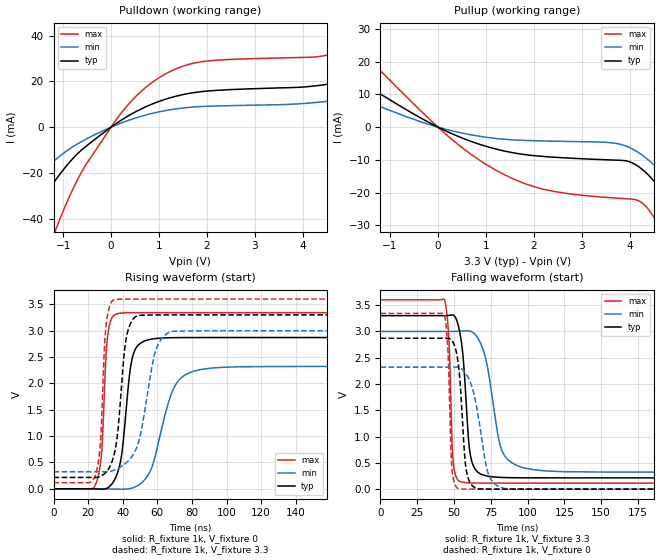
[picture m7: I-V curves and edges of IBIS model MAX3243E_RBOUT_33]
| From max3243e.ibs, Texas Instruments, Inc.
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[Model]   MAX3243E_RBOUT_33
Model_type  Output
Vref =   0
Rref =   3000
Cref =   150p
Vmeas =   1.5
| variable   typ   min   max
C_comp   4.21pF   3.18pF   6.18pF
| C_pullup   3.97pF   3.18pF   5.18pF
| C_pulldown   4.44pF   3.29pF   6.18pF
[Temperature Range]   40   100   -40
| Ambient temperature   25   85   -40
[Voltage range]   3.3   3   3.6
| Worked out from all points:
|   slope of the pulldown table from 0 to 0.495 V, typ, clamps not added: 75.9 ohm
|   slope of the pullup table from 0 to 0.495 V, typ, clamps not added: 152 ohm
|   rising waveform, R_fixture 1k, V_fixture 0: 20-80 % time 5.45ns typ, 11.3ns min, 2.9ns max; typ from 0 V to 2.87 V
|   falling waveform, R_fixture 1k, V_fixture 3.3: 20-80 % time 4.69ns typ, 9.47ns min, 2.43ns max; typ from 3.3 V to 0.215 V
|   rising waveform, R_fixture 1k, V_fixture 3.3: 20-80 % time 5.08ns typ, 8.91ns min, 2.91ns max; typ from 0.215 V to 3.3 V
|   falling waveform, R_fixture 1k, V_fixture 0: 20-80 % time 4.16ns typ, 8.6ns min, 2.22ns max; typ from 2.87 V to 0 V
[Pulldown]
| MAX3243E_RBOUT_33
|   Voltage   I(typ)   I(min)   I(max)
-3.3V     -113.4mA   -74.18mA   -190mA
-2.415V   -70.58mA   -44.83mA   -126.3mA
-1.81V    -45.3mA    -28.2mA    -84.59mA
-1.175V   -23.63mA   -14.52mA   -45.99mA
-595mV    -9.62mA    -6.087mA   -18.88mA
200mV     2.877mA    1.713mA    5.857mA
705mV     8.707mA    5.186mA    17.04mA
1.335V    13.41mA    7.923mA    25.3mA
2.01V     15.77mA    9.121mA    28.89mA
4.405V    18.41mA    11.05mA    31.05mA
6.135V    26.75mA    17.02mA    43.3mA
6.6V      29.92mA    19.27mA    48.02mA
[Pullup]
| MAX3243E_RBOUT_33
|   Voltage   I(typ)   I(min)   I(max)
-3.3V     30.08mA    19.81mA    47.96mA
-2.18V    19.23mA    12.28mA    31.63mA
335mV     -2.284mA   -1.265mA   -4.285mA
1.66V     -8.06mA    -3.97mA    -16.36mA
2.54V     -9.29mA    -4.322mA   -19.92mA
3.89V     -10.22mA   -5.614mA   -21.83mA
4.205V    -12.28mA   -7.993mA   -22.63mA
4.46V     -15.74mA   -10.94mA   -26.56mA
4.625V    -18.71mA   -13.31mA   -30.76mA
5.14V     -31.25mA   -22.85mA   -49.93mA
5.47V     -41.58mA   -30.54mA   -65.91mA
6.6V      -87.28mA   -64.61mA   -134mA
[Ramp]
| MAX3243E_RBOUT_33
| variable   typ   min   max
dV/dt_r   1.73/5.46E-09   1.40/1.14E-08   2.01/2.91E-09
dV/dt_f   1.86/4.72E-09   1.61/9.50E-09   2.10/2.45E-09
R_load = 1k
[Rising Waveform]
| MAX3243E_RBOUT_33
R_fixture =   1k
C_fixture =   0
L_fixture =   0
V_fixture =   0
V_fixture_min = 0
V_fixture_max = 0
|   Time   V(typ)   V(min)   V(max)
0s        331.6pV    2.084nV    131.1pV
24.9ns    -3.34mV    12.77uV    132.3mV
27.9ns    -6.992mV   80.13uV    738.9mV
31.2ns    16.85mV    -1.213mV   2.874V
36.2ns    234.8mV    -5.782mV   3.314V
45.3ns    2.449V     12.87mV    3.341V
53.4ns    2.814V     200.5mV    3.342V
69.2ns    2.867V     1.889V     3.342V
81.2ns    2.87V      2.233V     3.342V
269.9ns   2.87V      2.321V     3.342V
[Falling Waveform]
| MAX3243E_RBOUT_33
R_fixture =   1k
C_fixture =   0
L_fixture =   0
V_fixture =   3.3
V_fixture_min = 3
V_fixture_max = 3.6
|   Time   V(typ)   V(min)   V(max)
0s        3.3V       3V         3.6V
43.6ns    3.3V       3V         3.597V
46.5ns    3.305V     3V         2.86V
49.4ns    3.311V     3V         551.1mV
53.9ns    2.994V     3.004V     147.3mV
60.9ns    691mV      3.005V     119mV
68.2ns    288.3mV    2.768V     115.8mV
81.6ns    224mV      815.7mV    115.3mV
92.9ns    217mV      449.6mV    115.2mV
269.9ns   215.4mV    323.9mV    115.2mV
[Rising Waveform]
| MAX3243E_RBOUT_33
R_fixture =   1k
C_fixture =   0
L_fixture =   0
V_fixture =   3.3
V_fixture_min = 3
V_fixture_max = 3.6
|   Time   V(typ)   V(min)   V(max)
0s        215.4mV    323.9mV    115.2mV
24.2ns    214.5mV    323.9mV    264.1mV
27.1ns    238.6mV    323.8mV    885.1mV
30.3ns    309.9mV    323mV      3.075V
34.7ns    609.5mV    349mV      3.582V
41.9ns    2.831V     489.1mV    3.599V
48.4ns    3.283V     810.2mV    3.6V
58.7ns    3.299V     2.58V      3.6V
67.7ns    3.3V       2.978V     3.6V
269.9ns   3.3V       3V         3.6V
[Falling Waveform]
| MAX3243E_RBOUT_33
R_fixture =   1k
C_fixture =   0
L_fixture =   0
V_fixture =   0
V_fixture_min = 0
V_fixture_max = 0
|   Time   V(typ)   V(min)   V(max)
0s        2.87V      2.321V     3.342V
43.3ns    2.871V     2.321V     3.316V
45.9ns    2.87V      2.321V     2.634V
48.6ns    2.825V     2.322V     399mV
53ns      2.369V     2.319V     9.695mV
58.1ns    411.2mV    2.196V     1.125mV
65ns      18.23mV    1.622V     247.2uV
73ns      1.936mV    322.1mV    75.72uV
82.9ns    465.6uV    23.57mV    25.62uV
269.9ns   -1.212nV   7.853nV    -883pV
